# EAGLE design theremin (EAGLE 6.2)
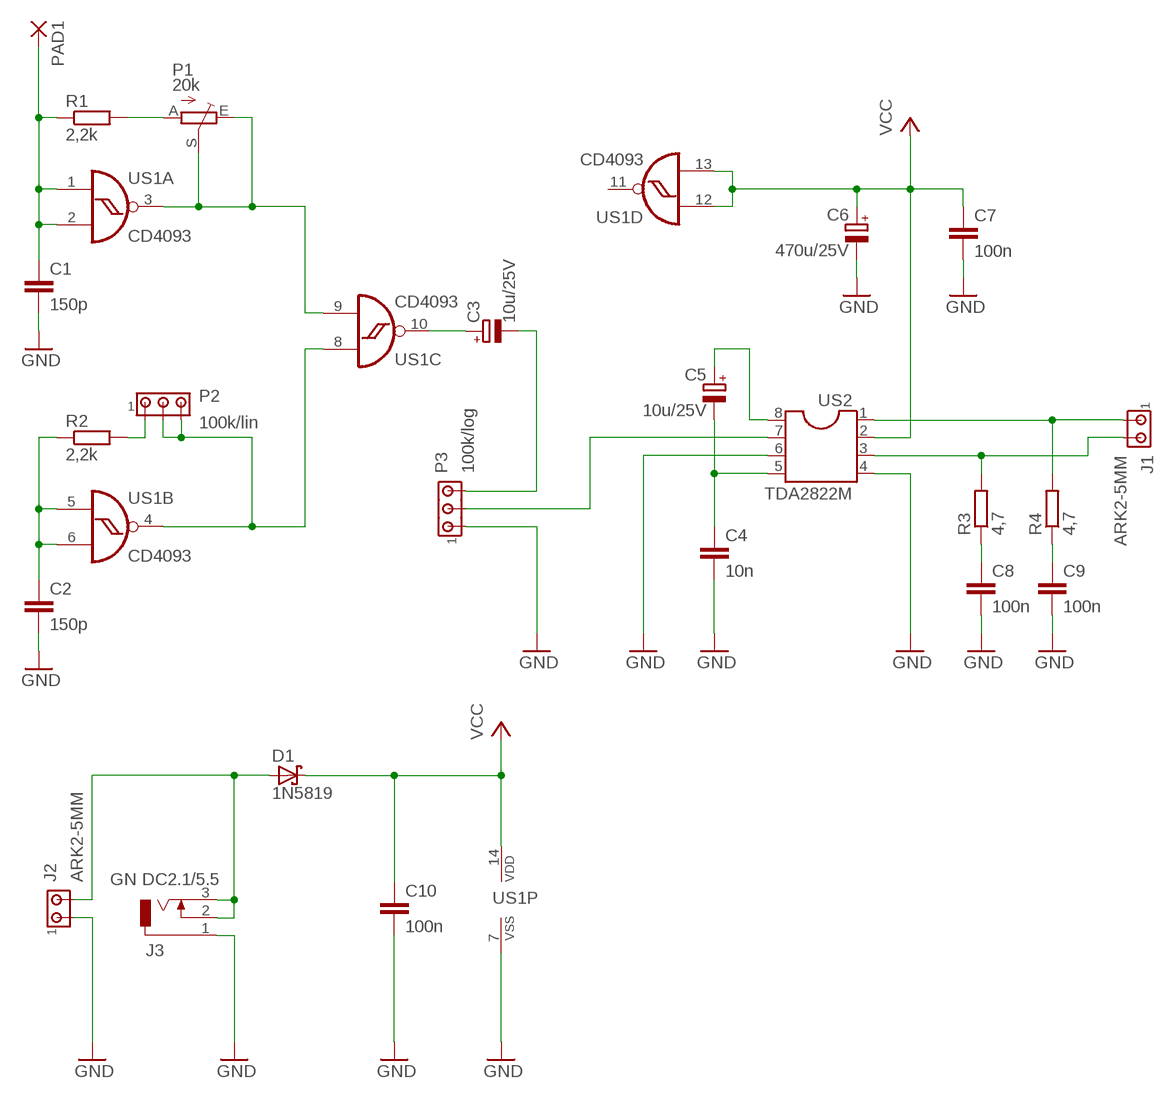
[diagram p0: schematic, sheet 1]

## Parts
C1  150p  C-EU050-025X075  [C050-025X075]
C2  150p  C-EU050-025X075  [C050-025X075]
C3  10u/25V  CPOL-EUE2.5-5  [E2,5-5]
C4  10n  C-EU050-025X075  [C050-025X075]
C5  10u/25V  CPOL-EUE2.5-5  [E2,5-5]
C6  470u/25V  CPOL-EUE3.5-8  [E3,5-8]
C7  100n  C-EU050-025X075  [C050-025X075]
C8  100n  C-EU050-025X075  [C050-025X075]
C9  100n  C-EU050-025X075  [C050-025X075]
C10  100n  C-EU050-025X075  [C050-025X075]
D1  1N5819  1N5819-T  [DO41-7.6]
J1  ARK2-5MM  [2PIN-5MM]
J2  ARK2-5MM  [2PIN-5MM]
J3  GN DC2.1/5.5  DCJ0202  [DCJ0202]
P1  20k  TRIM_EU-CA6V  [CA6V]
P2  100k/lin  ARK3-5MM-WASKI  [3PIN-5M-WASKI]
P3  100k/log  ARK3-5MM-WASKI  [3PIN-5M-WASKI]
PAD1  WIREPAD2/4  [2/4]
R1  2,2k  R-EU_0207/7  [0207/7]
R2  2,2k  R-EU_0207/7  [0207/7]
R3  4,7  R-EU_0207/7  [0207/7]
R4  4,7  R-EU_0207/7  [0207/7]
US1  CD4093  4093N  [DIL14]
US2  TDA2822M  DIL8  [DIL08]

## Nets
GND: C1.2 C2.2 C4.2 C6.- C7.2 C8.2 C9.2 C10.2 J2.P$1 J3.1 P3.P$1 US1.7(P:VSS) US2.4 US2.6
N$1: C2.1 R2.1 US1.5(B:I0) US1.6(B:I1)
N$2: P2.P$2 P2.P$3 US1.4(B:O) US1.8(C:I0)
N$3: P2.P$1 R2.2
N$4: C1.1 PAD1.P$1(P) R1.1 US1.1(A:I0) US1.2(A:I1)
N$5: P1.A R1.2
N$6: P1.E P1.S US1.3(A:O) US1.9(C:I1)
N$7: C4.1 C5.- US2.5
N$8: C3.+ US1.10(C:O)
N$9: P3.P$2 US2.7
N$12: C5.+ US2.8
N$15: J1.P$2 R3.2 US2.3
N$16: C8.1 R3.1
N$17: J1.P$1 R4.2 US2.1
N$18: C9.1 R4.1
N$20: C3.- P3.P$3
N$38: D1.A J2.P$2 J3.2 J3.3
VCC: C6.+ C7.1 C10.1 D1.C US1.12(D:I0) US1.13(D:I1) US1.14(P:VDD) US2.2
Unconnected: US1.11(D:O)

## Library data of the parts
C1 C2 C4 C7-C10 = rcl:C-EU: CAPACITOR, European symbol
C3 C5 C6 = rcl:CPOL-EU: POLARIZED CAPACITOR, European symbol
D1 = diode:1N581*: 1.0A SCHOTTKY BARRIER RECTIFIER
J1 J2 = zlacza_futrzak:ARK2: ARK 2
J3 = con-jack:DCJ0202: DC POWER JACK Source: DCJ0202.pdf; OC_FARNELL: unknown; OC_NEWARK: unknown
P1 = pot:TRIM_EU-: POTENTIOMETER
P2 P3 = zlacza_futrzak:ARK3: ARK 3 Raster 5mm i 3,5mm
PAD1 = zlacza_futrzak:WIREPAD
R1-R4 = rcl:R-EU_: RESISTOR, European symbol
US1 = 40xx:4093: Quad 2-input NAND schmitt trigger
US2 = ic-package:DIL8: Dual In Line / Socket

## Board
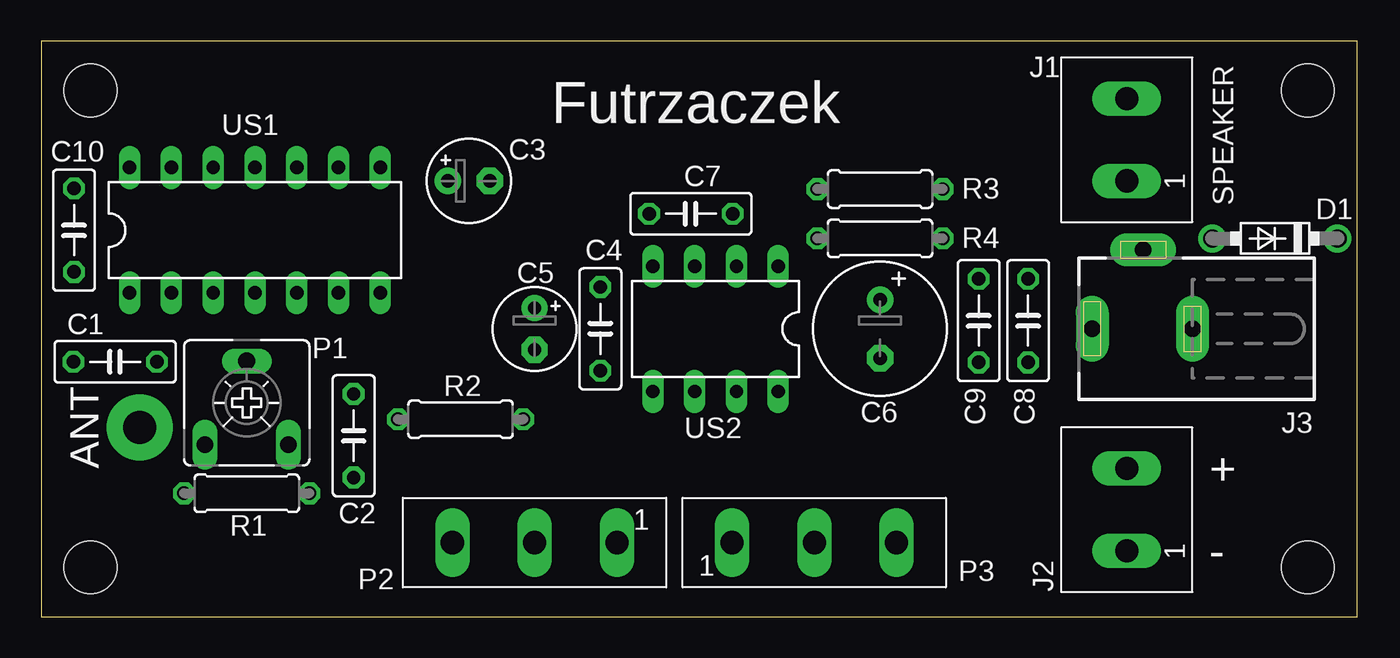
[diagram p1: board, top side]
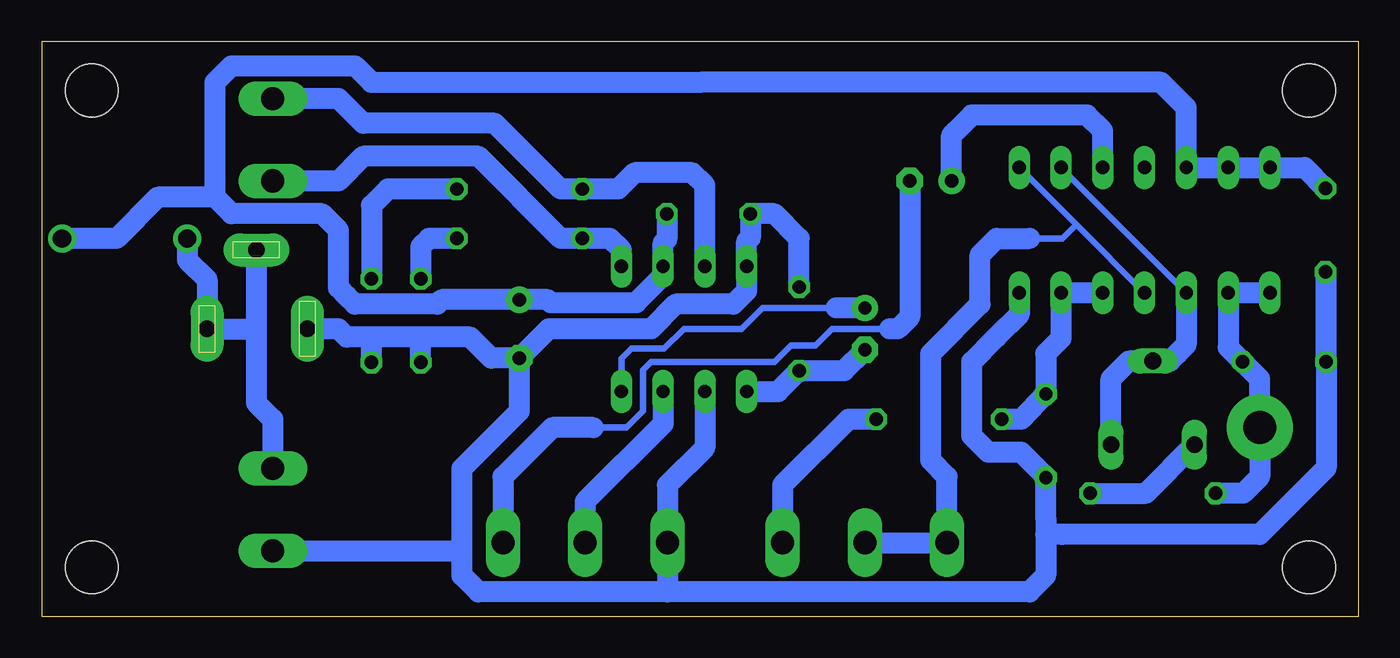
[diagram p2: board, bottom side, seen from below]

Size 80 x 35 mm. Coordinates in mm from the lower left corner, seen from the top.
Outline: 0,0 80,0 80,35 0,35 0,0
Copper layers (1*16): Top 0.035mm / dielectric 1.5mm / Bottom 0.035mm
Design rules: minimum track width 10mil, minimum drill 24mil, track to track 8mil, track to pad 8mil, pad to pad 8mil, via to via 8mil, smd to smd 8mil, copper to edge 20mil, drill to drill 8mil, minimum pad ring 10mil, minimum via ring 8mil, stop-mask expansion 4mil, vias tented up to drill 0mil, thermal gap 10mil
Holes 3.2 mm at 3,3 3,32 77,3 77,32

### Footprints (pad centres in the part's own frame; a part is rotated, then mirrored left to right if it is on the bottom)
C050-025X075 = drill 0.813 octagon: 1 -2.54,0; 2 2.54,0
E2,5-5 = drill 0.813 pad 1.6: + -1.27,0 | drill 0.813 pad 1.6 octagon: - 1.27,0
E3,5-8 = drill 0.813 pad 1.6: + -1.778,0 | drill 0.813 pad 1.6 octagon: - 1.778,0
DO41-7.6 = drill 1.1 pad 1.7: A 3.81,0; C -3.81,0
2PIN-5MM = drill 1.4 long: P$1 -2.5,0; P$2 2.5,0
DCJ0202 = drill 1 pad 2 long: 1 0,3.1; 2 4.8,0; 3 0,-3
CA6V = drill 1.016 long: A -2.54,-2.54; E 2.54,-2.54; S 0,2.54
3PIN-5M-WASKI = drill 1.4 long: P$1 -5,0; P$2 0,0; P$3 5,0
2/4 = drill 2 pad 4: P$1 0,0
0207/7 = drill 0.813 octagon: 1 -3.81,0; 2 3.81,0
DIL14 = drill 0.813 long: 1 -7.62,-3.81; 2 -5.08,-3.81; 3 -2.54,-3.81; 4 0,-3.81; 5 2.54,-3.81; 6 5.08,-3.81; 7 7.62,-3.81; 8 7.62,3.81; 9 5.08,3.81; 10 2.54,3.81; 11 0,3.81; 12 -2.54,3.81; 13 -5.08,3.81; 14 -7.62,3.81
DIL08 = drill 0.813 long: 1 -3.81,-3.81; 2 -1.27,-3.81; 3 1.27,-3.81; 4 3.81,-3.81; 5 3.81,3.81; 6 1.27,3.81; 7 -1.27,3.81; 8 -3.81,3.81

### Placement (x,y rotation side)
C1  4.5,15.5 180 top
C2  19,11 270 top
C3  26,26.5 0 top
C4  34,17.5 90 top
C5  30,17.5 270 top
C6  51,17.5 270 top
C7  39.5,24.5 180 top
C8  60,18 270 top
C9  57,18 270 top
C10  2,23.5 270 top
D1  75,23 180 top
J1  66,29 90 top
J2  66,6.5 90 top
J3  67,17.5 90 top
P1  12.5,13 0 top
P2  30,4.5 180 top
P3  47,4.5 0 top
PAD1  6,11.5 0 top
R1  12.5,7.5 0 top
R2  25.5,12 0 top
R3  51,26 180 top
R4  51,23 180 top
US1  13,23.5 0 top
US2  41,17.5 180 top

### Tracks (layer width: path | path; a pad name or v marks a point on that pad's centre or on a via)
GND
  Bottom 1.27: US1.7 20.62,18.38 22,17 23.5,15.5 23.5,11 22.5,10 20.5,10 19,8.5 C2.2 19,6 19,5 | C10.2 1.96,20.92 C1.2 1.96,9.04 6,5 18,5 19,5 | 19,5 19,2.5 20,1.5 42,1.5 | 42,1.5 P3.P$1 42,8 39.73,10.27 US2.6 | 42,1.5 53.5,1.5 54.5,2.5 54.5,4 | 54.5,4 54.5,9 51,12.5 C6.- | C4.2 34,23 35.5,24.5 C7.2 36.96,23.04 37,23 37.19,22.81 US2.4 37.19,19.81 38,19 41.5,19 43,17.5 49.22,17.5 C6.- | J2.P$1 54.5,4 | C6.- 52.72,15.72 54,17 57,17 | 57,17 60,17 | 60,17 61.5,17 62,17.5 J3.1 | C8.2 60,17 | C9.2 57,17
N$1
  Bottom 1.27: US1.5 US1.6 18.08,16.92 19,16 C2.1 19.04,13.54 20.5,12 R2.1
N$2
  Bottom 0.406: US1.4 17.16,23.84 | 17.16,23.84 US1.8 | 20,23 18,23 17.16,23.84
  Bottom 1.27: P2.P$2 P2.P$3 25,8.5 26,9.5 26,16 23,19 23,22 22,23 20,23
N$3
  Bottom 1.27: R2.2 31,12 35,8 P2.P$1
N$4
  Bottom 1.27: US1.1 US1.2 7.92,16.38 C1.1 6,14.46 PAD1.P$1 6,8.5 7,7.5 R1.1
N$5
  Bottom 1.27: R1.2 12.92,7.5 P1.A
N$6
  Bottom 0.406: US1.3 US1.9
  Bottom 1.27: US1.3 10.46,16.54 11,16 11.46,15.54 P1.S 13.96,15.54 14.5,15 15.04,14.46 P1.E
N$7
  Bottom 1.27: US2.5 35.27,13.69 C4.1 31.27,14.96 C5.-
N$8
  Bottom 1.27: US1.10 15.54,29.54 16.5,30.5 23.5,30.5 24.5,29.5 24.73,29.27 C3.+
N$9
  Bottom 1.27: US2.7 42.27,11.73 47,7 P3.P$2
N$12
  Bottom 0.406: 31.73,18.77 36.23,18.77 37.5,17.5 41,17.5 42.2,16.3 44.2,16.3 44.81,15.69 US2.8
  Bottom 1.27: C5.+ 31.73,18.77
N$15
  Bottom 1.27: US2.3 39.73,26.23 40.5,27 44,27 45,26 R3.2 48.5,26 52.5,30 60.5,30 62,31.5 J1.P$2
N$16
  Bottom 1.27: R3.1 59,26 60,25 C8.1
N$17
  Bottom 1.27: US2.1 44.81,22.31 45.5,23 R4.2 48.5,23 53.5,28 60.5,28 62,26.5 J1.P$1
N$18
  Bottom 1.27: R4.1 56.5,23 57,22.5 C9.1
N$20
  Bottom 0.406: 28.5,17.5 32,17.5 33,16.5 34.5,16.5 35.5,15.5 43,15.5 43.5,15 43.5,12.5 44.5,11.5 46.5,11.5
  Bottom 1.27: C3.- 27.27,18.23 28,17.5 28.5,17.5 | 46.5,11.5 49,11.5 52,8.5 P3.P$3
N$38
  Bottom 1.27: J3.2 67,17.5 | 67,17.5 67,13 66,12 J2.P$2 | J3.3 69.5,17.5 | 69.5,17.5 67,17.5 | 69.5,17.5 70,18 70,20.5 71.19,21.69 D1.A
VCC
  Bottom 1.27: C10.1 3.27,27.31 US1.14 US1.13 US1.12 10.46,30.96 12,32.5 40,32.5 60,32.5 61,33.5 68.5,33.5 69.5,32.5 69.5,25.5 | C7.1 42.04,22.96 42.27,22.73 US2.2 42.27,20.73 43.9,19.1 49.1,19.1 49.28,19.28 C6.+ 55.72,19.28 56,19 61,19 61.5,19.5 62,20 62,23.5 63,24.5 68.5,24.5 69.5,25.5 | 69.5,25.5 73,25.5 75.5,23 D1.C

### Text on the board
tPlace: Futrzaczek | SPEAKER | ANT | + | -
